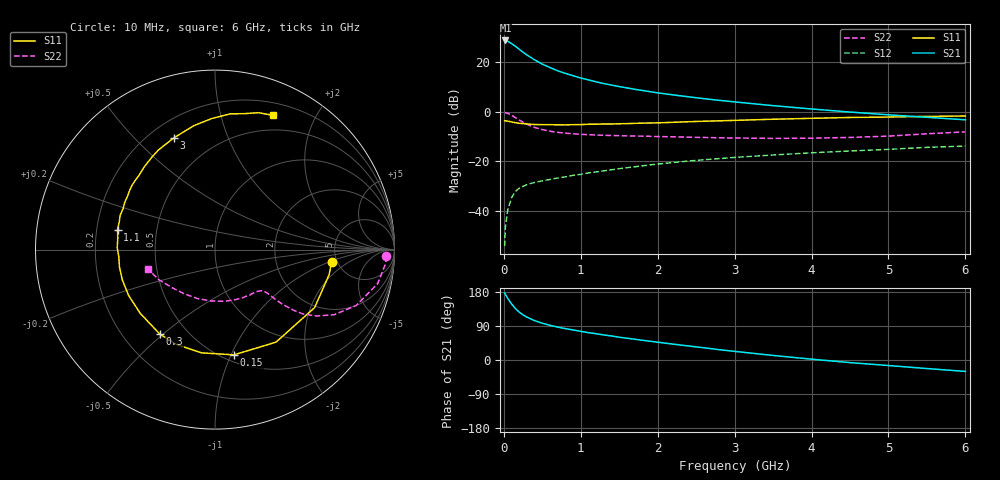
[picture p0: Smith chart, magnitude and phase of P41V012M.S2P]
! SIEMENS Small Signal Semiconductors
! BFP182
! Si NPN RF Bipolar Junction Transistor in SOT143
! VCE = 1 V  IC = 12 mA
! Common Emitter S-Parameters:  March  1996
# GHz  S  MA  R  50
!  f  S11  S21  S12  S22
! GHz  MAG  ANG  MAG  ANG  MAG  ANG  MAG  ANG
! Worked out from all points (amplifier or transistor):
!   36 points, 10 MHz to 6 GHz, reference 50 ohm
!   highest |S21| = 28.8 dB at 20 MHz (marker M1)
!   |S21| within 3 dB of that: start of sweep to 177.3 MHz
!   unconditionally stable (mu >= 1): 755.1 MHz to end of sweep
!   at 250 MHz: K = 0.44, MSG = 27.1 dB, |S12| = -30.2 dB
!   at 1.4 GHz: K = 1.27, MAG = 14.0 dB, |S12| = -23.5 dB
!   at 6 GHz: K = 1.05, MAG = 3.9 dB, |S12| = -14.0 dB
!   S11 on the Smith chart (normalised r, x): 10 MHz: 4.49, -1.09; 150 MHz: 0.56, -1.03; 300 MHz: 0.35, -0.49; 1.1 GHz: 0.29, +0.09; 3 GHz: 0.30, +0.66; 6 GHz: 0.33, +1.47
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0.01  0.6534 -6.1  27.23 176.7  0.0019 74.5  0.9557 -2.3
0.02  0.651 -12.4  27.44 173.5  0.0046 80.7  0.9532 -4.8
0.05  0.6422 -30.2  26.52 162.9  0.0101 79.4  0.9259 -11.8
0.1  0.6176 -56.6  23.8 148.1  0.0181 63.5  0.8461 -21.6
0.15  0.5959 -79.8  20.93 135.7  0.0243 55.9  0.7559 -28.7
0.2  0.5801 -97.4  18.25 126.4  0.0282 51.6  0.6755 -33.2
0.25  0.5708 -111.8  15.83 118.9  0.0308 47.1  0.6078 -36.2
0.3  0.5623 -123.1  13.97 113.1  0.0334 45.1  0.5525 -37.7
0.4  0.5475 -139.5  11.12 103.8  0.0369 42.8  0.4783 -39.1
0.5  0.545 -152.0  9.117 97.1  0.0398 42.0  0.4321 -39.5
0.6  0.5432 -161.8  7.765 91.5  0.0425 42.6  0.4014 -39.6
0.7  0.5412 -169.5  6.682 86.9  0.0454 43.1  0.381 -39.7
0.8  0.5376 -175.9  5.924 82.8  0.048 43.7  0.3662 -40.1
1  0.5454 173.3  4.776 75.7  0.0538 45.1  0.3474 -41.2
1.1  0.5545 168.4  4.37 72.2  0.0576 45.2  0.3414 -42.3
1.5  0.5672 152.6  3.207 60.1  0.0702 45.9  0.3259 -47.4
2.2  0.6071 130.3  2.176 41.9  0.0933 43.2  0.3092 -60.4
3  0.6639 110.0  1.571 22.8  0.1185 37.9  0.2923 -80.2
3.5  0.7008 99.6  1.318 12.0  0.1326 33.7  0.2872 -94.6
4.5  0.7609 83.6  0.979 -6.9  0.1599 25.5  0.3001 -124.9
5.5  0.8002 72.4  0.766 -22.6  0.1893 17.4  0.3561 -152.0
6  0.8145 66.7  0.683 -30.1  0.2005 12.5  0.3892 -164.0
